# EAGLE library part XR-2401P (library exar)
MICROCONTROLLER
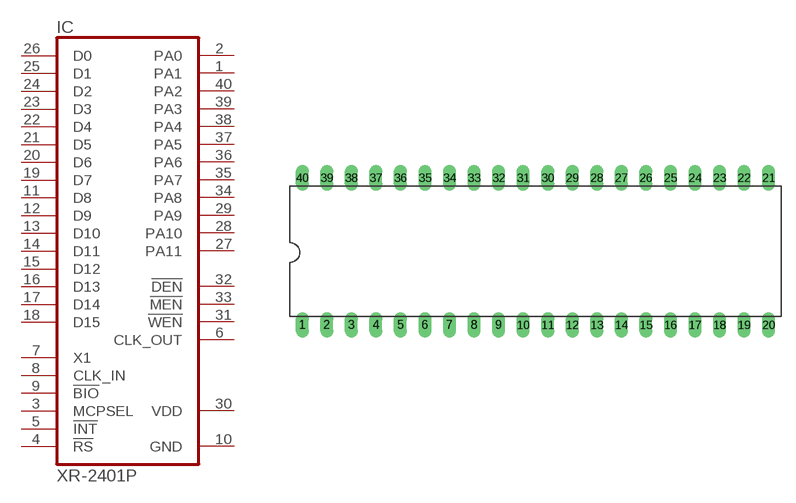
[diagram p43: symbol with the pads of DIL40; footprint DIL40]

Designator prefix IC

## XR-2401P (OC_FARNELL: unknown; OC_NEWARK: unknown)  [DIL40]
1  PA1  out
2  PA0  out
3  MCPSEL  in
4  !RS  in
5  !INT  in
6  CLK_OUT  out
7  X1  in
8  CLK_IN  in
9  !BIO  in
10  GND  pwr
11  D8
12  D9
13  D10
14  D11
15  D12
16  D13
17  D14
18  D15
19  D7
20  D6
21  D5
22  D4
23  D3
24  D2
25  D1
26  D0
27  PA11  out
28  PA10  out
29  PA9  out
30  VDD  pwr
31  !WEN  out
32  !DEN  out
33  !MEN  out
34  PA8  out
35  PA7  out
36  PA6  out
37  PA5  out
38  PA4  out
39  PA3  out
40  PA2  out

## Footprint DIL40 (pad centres in mm)
Dual In Line Package
drill 0.813 long: 1 -24.13,-7.62; 2 -21.59,-7.62; 3 -19.05,-7.62; 4 -16.51,-7.62; 5 -13.97,-7.62; 6 -11.43,-7.62; 7 -8.89,-7.62; 8 -6.35,-7.62; 9 -3.81,-7.62; 10 -1.27,-7.62; 11 1.27,-7.62; 12 3.81,-7.62; 13 6.35,-7.62; 14 8.89,-7.62; 15 11.43,-7.62; 16 13.97,-7.62; 17 16.51,-7.62; 18 19.05,-7.62; 19 21.59,-7.62; 20 24.13,-7.62; 21 24.13,7.62; 22 21.59,7.62; 23 19.05,7.62; 24 16.51,7.62; 25 13.97,7.62; 26 11.43,7.62; 27 8.89,7.62; 28 6.35,7.62; 29 3.81,7.62; 30 1.27,7.62; 31 -1.27,7.62; 32 -3.81,7.62; 33 -6.35,7.62; 34 -8.89,7.62; 35 -11.43,7.62; 36 -13.97,7.62; 37 -16.51,7.62; 38 -19.05,7.62; 39 -21.59,7.62; 40 -24.13,7.62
